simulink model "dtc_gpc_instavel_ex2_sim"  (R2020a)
settings: Solver=VariableStepAuto  StartTime=0.0  StopTime=tsim  MaxStep=0.01  RelTol=1e-3
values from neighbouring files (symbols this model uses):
  amppert = 0.05    [dtc_gpc_temperatura.m]    (also in dtc_gpc_instavel_ex_2.m = 0)
  ampref = 0.5    [dtc_gpc_temperatura.m]    (also in dtc_gpc_instavel_ex_2.m = 0.6)
  Fdtc = Ftemp    [dtc_gpc_temperatura.m]    (also in dtc_gpc_instavel_ex_2.m)
  Hdtc = cell2mat(H)    [dtc_gpc_temperatura.m]    (also in dtc_gpc_instavel_ex_2.m)
  Kdtc1 = [Kdtc1; Kdtc(sum(Nu(1:i-1))+1,:)]    [dtc_gpc_temperatura.m]    (also in dtc_gpc_instavel_ex_2.m)
  tpert = 20    [dtc_gpc_temperatura.m]    (also in dtc_gpc_instavel_ex_2.m = 30)
  tref = 2    [dtc_gpc_temperatura.m]    (also in dtc_gpc_instavel_ex_2.m = 5)
  Ts = 0.2    [dtc_gpc_temperatura.m]    (also in trocador_PS_GPC_dtc.m = 0.15; dtc_gpc_instavel_exemplo_1.m = 1; dtc_mimo_ex1.m = 1; dtc_gpc_instavel_ex_2.m = 1)
  zr_dtc = blkdiag(zr_dtc,ones(Ny(i),1))    [dtc_gpc_temperatura.m]    (also in dtc_gpc_instavel_ex_2.m)
libraries: cstblocks x5

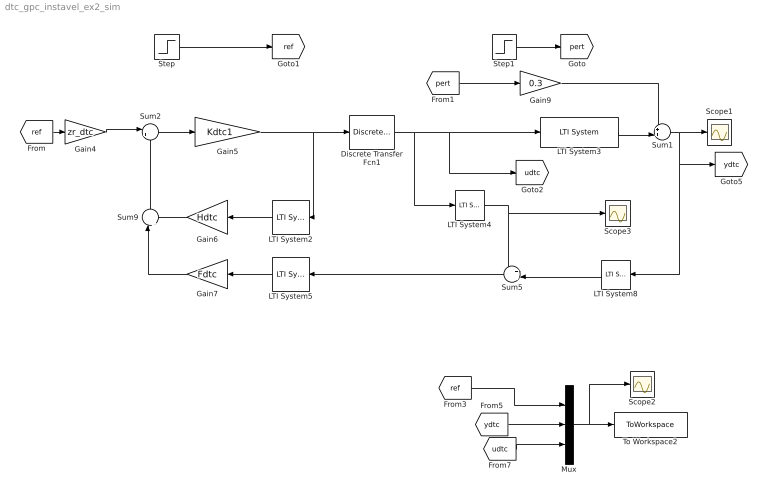
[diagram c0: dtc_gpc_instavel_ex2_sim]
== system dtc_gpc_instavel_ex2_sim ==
  Discrete Transfer Fcn1 : DiscreteTransferFcn  Numerator=[1 0]  Denominator=[1 -1]  SampleTime=Ts
  Gain4 : Gain  Gain=zr_dtc  Multiplication=Matrix(K*u)
  Gain5 : Gain  Gain=Kdtc1  Multiplication=Matrix(K*u)
  Gain6 : Gain  Gain=Hdtc  Multiplication=Matrix(K*u)
  Gain7 : Gain  Gain=Fdtc  Multiplication=Matrix(K*u)
  Gain9 : Gain  Gain=0.3  Multiplication=Matrix(K*u)
  LTI System2 : cstblocks/LTI System  sys=zu_dtc  IC=[]
  LTI System3 : cstblocks/LTI System  sys=P  IC=[]
  LTI System4 : cstblocks/LTI System  sys=S  IC=[]
  LTI System5 : cstblocks/LTI System  sys=zy_dtc  IC=[]
  LTI System8 : cstblocks/LTI System  sys=Fe  IC=[]
  Mux : Mux  Inputs=3
  Scope1 : Scope
  Scope2 : Scope
  Scope3 : Scope
  Step : Step  Time=tref  After=ampref  SampleTime=0
  Step1 : Step  Time=tpert  After=amppert  SampleTime=0
  Sum1 : Sum  Inputs=++|
  Sum2 : Sum  Inputs=|+-
  Sum5 : Sum  Inputs=++|
  Sum9 : Sum  Inputs=|++
  To Workspace2 : ToWorkspace  VariableName=simout  SampleTime=-1
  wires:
  Step/1 -> [ref]
  LTI System4/1 -> Sum5/1, Scope3/1
  Sum1/1 -> LTI System8/1, [ydtc], Scope1/1
  Mux/1 -> Scope2/1, To Workspace2/1
  [ref] -> Mux/1
  LTI System8/1 -> Sum5/2
  Gain6/1 -> Sum9/2
  LTI System5/1 -> Gain7/1
  LTI System2/1 -> Gain6/1
  Gain7/1 -> Sum9/1
  [ref] -> Gain4/1
  Gain5/1 -> LTI System2/1, Discrete Transfer Fcn1/1
  Gain4/1 -> Sum2/1
  Sum9/1 -> Sum2/2
  Sum2/1 -> Gain5/1
  Sum5/1 -> LTI System5/1
  Step1/1 -> [pert]
  Discrete Transfer Fcn1/1 -> LTI System3/1, [udtc], LTI System4/1
  Gain9/1 -> Sum1/1
  LTI System3/1 -> Sum1/2
  [pert] -> Gain9/1
  [ydtc] -> Mux/2
  [udtc] -> Mux/3
